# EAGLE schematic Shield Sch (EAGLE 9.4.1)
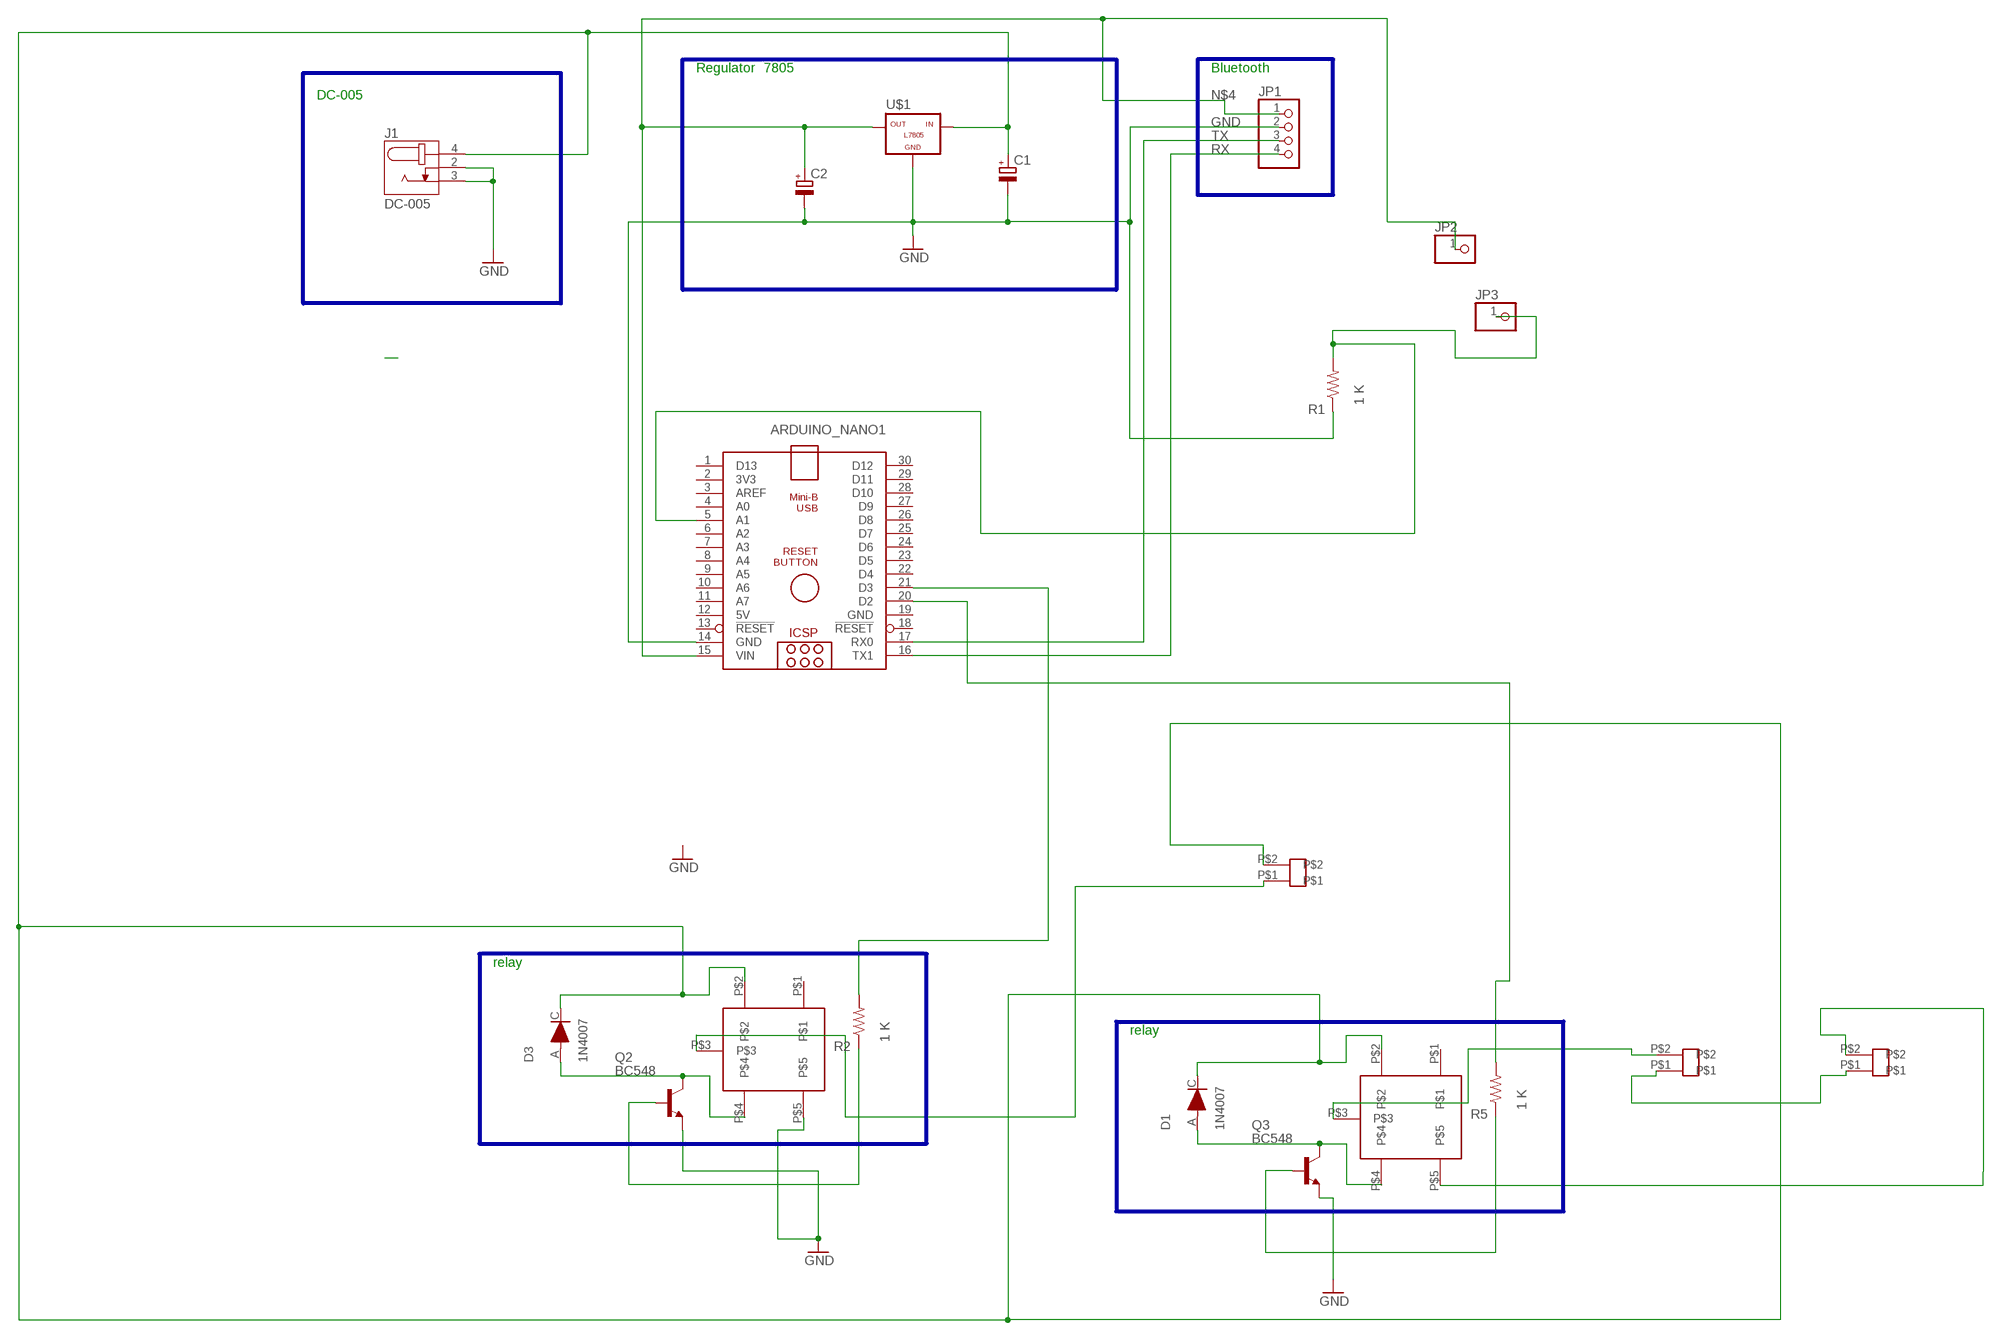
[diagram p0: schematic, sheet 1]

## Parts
ARDUINO_NANO1  ARDUINO_NANO  [ARDUINO_NANO]
C1  CPOL-EUE2.5-6  [E2,5-6]
C2  CPOL-EUE2.5-6  [E2,5-6]
D1  1N4007  [DIOAD1060W80L520D270]
D3  1N4007  [DIOAD1060W80L520D270]
J1  DC-005  [NINIGI_DC-005]
JP1  PINHD-1X4  [1X04]
JP2  PINHD-1X1  [1X01]
JP3  PINHD-1X1  [1X01]
Q2  BC548  [TO92-EBC]
Q3  BC548  [TO92-EBC]
R1  1 K  RES-US1206FAB  [R1206FAB]
R2  1 K  RES-US1206FAB  [R1206FAB]
R5  1 K  RES-US1206FAB  [R1206FAB]
U$1  -L7805  [L7805]
U$3  RELAYSL  [RELAYSL]
U$5  RELAYSL  [RELAYSL]
U$6  CNN  [CNN]
U$7  CNN  [CNN]
U$8  CNN  [CNN]

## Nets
GND: ARDUINO_NANO1.14(GND) C1.- C2.- J1.2 J1.3 JP1.2 Q2.E Q3.E R1.1 U$1.GND U$3.P$5
N$3: D3.A Q2.C U$3.P$4
N$4: ARDUINO_NANO1.15(VIN) C2.+ JP1.1 JP2.1 U$1.OUT
N$5: ARDUINO_NANO1.5(A1) JP3.1 R1.2
N$6: Q2.B R2.1
N$8: ARDUINO_NANO1.21(D3) R2.2
N$9: D1.A Q3.C U$5.P$4
N$11: Q3.B R5.1
N$12: ARDUINO_NANO1.20(D2) R5.2
N$14: U$5.P$3 U$7.P$2
N$15: U$6.P$1 U$7.P$1
N$16: U$3.P$3 U$8.P$1
N$17: U$5.P$5 U$6.P$2
RX: ARDUINO_NANO1.16(TX1) JP1.4
TX: ARDUINO_NANO1.17(RX0) JP1.3
VCC: C1.+ D1.C D3.C J1.4 U$1.IN U$3.P$2 U$5.P$2 U$8.P$2
Unconnected: ARDUINO_NANO1.1(D13) ARDUINO_NANO1.2(3V3) ARDUINO_NANO1.3(AREF) ARDUINO_NANO1.4(A0) ARDUINO_NANO1.6(A2) ARDUINO_NANO1.7(A3) ARDUINO_NANO1.8(A4) ARDUINO_NANO1.9(A5) ARDUINO_NANO1.10(A6) ARDUINO_NANO1.11(A7) ARDUINO_NANO1.13(!RESET) ARDUINO_NANO1.18(!RESET) ARDUINO_NANO1.22(D4) ARDUINO_NANO1.23(D5) ARDUINO_NANO1.24(D6) ARDUINO_NANO1.25(D7) ARDUINO_NANO1.26(D8) ARDUINO_NANO1.27(D9) ARDUINO_NANO1.28(D10) ARDUINO_NANO1.29(D11) ARDUINO_NANO1.30(D12) U$3.P$1 U$5.P$1

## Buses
B$5
7805/REGULATOR
B$1
B$2

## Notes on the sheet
- Regulator | 7805 | Bluetooth
- DC-005
- relay
- relay

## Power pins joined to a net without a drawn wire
5V: ARDUINO_NANO1.12(5V)
GND: ARDUINO_NANO1.19(GND)

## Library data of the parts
ARDUINO_NANO1 = ArduinoNanoV30:ARDUINO_NANO: Arduino Nano V3.0 Overview: The Arduino Nano is a small, complete, and breadboard-friendly board based on the ATmega328 (Arduino Nano 3.x) or ATmega168 (Arduino Nano 2.x). It has more or less the same functionality of the Arduino Duemilanove, but in a different package. It lacks only a DC power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
C1 C2 = Clean-Kong:CPOL-EU: POLARIZED CAPACITOR, European symbol
D1 D3 = 1N4007:1N4007: 1 Amp Rectifier; AVAILABILITY: Unavailable; DESCRIPTION: Diode, Standard Recovery, 1a, 1kv, Do-41, Full Reel; MF: Diodes; MP: 1N4007-T; PACKAGE: DO-41 Multicomp; PRICE: None
J1 = DC-005:DC-005: DC Jack; AVAILABILITY: Unavailable; MF: Littelfuse Inc.; MP: DC-005; PACKAGE: 0603 Ninigi; PRICE: None
JP1 = pinhead:PINHD-1X4: PIN HEADER
JP2 JP3 = pinhead:PINHD-1X1: PIN HEADER
Q2 Q3 = transistor-npn:BC548*: NPN Transistor
R1 R2 R5 = fab:RES-US: Resistor (US Symbol)
U$1 = tango:-L7805
U$3 U$5 = relay:RELAYSL
U$6-U$8 = resistor-bourns:CNN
